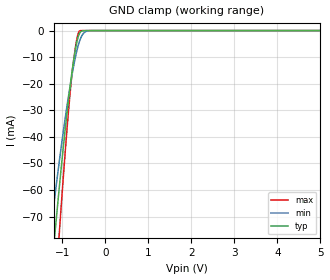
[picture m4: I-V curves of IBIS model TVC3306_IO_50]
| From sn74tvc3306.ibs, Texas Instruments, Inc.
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[Model]   TVC3306_IO_50
Model_type  Terminator
| variable   typ   min   max
C_comp   2.54pF   2.12pF   3.20pF
| C_tri-state   2.54pF   2.12pF   3.20pF
[Temperature Range]   40   100   -40
| Ambient temperature   25   85   -40
[Voltage range]   5   5   5
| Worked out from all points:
|   GND clamp passes 1 mA (typ) near -0.59 V on its own axis
[GND Clamp]
| TVC3306_IO_50
|   Voltage   I(typ)   I(min)   I(max)
-5V       -931.9mA   -737mA     -1.229A
-1.305V   -101.3mA   -80.91mA   -134.8mA
-1.26V    -93.01mA   -74.68mA   -123.4mA
-1.175V   -77.75mA   -63.23mA   -102.3mA
-1.06V    -58.02mA   -48.48mA   -74.88mA
-905mV    -33.62mA   -30.32mA   -40.74mA
-795mV    -18.51mA   -18.98mA   -20.12mA
-680mV    -6.109mA   -9.157mA   -5.225mA
-595mV    -1.038mA   -3.966mA   -104uA
-485mV    -31.54uA   -706.8uA   -862.7nA
-330mV    -244.7nA   -17.7uA    -1.795nA
5V        54.17pA    2.924nA    25.8pA
